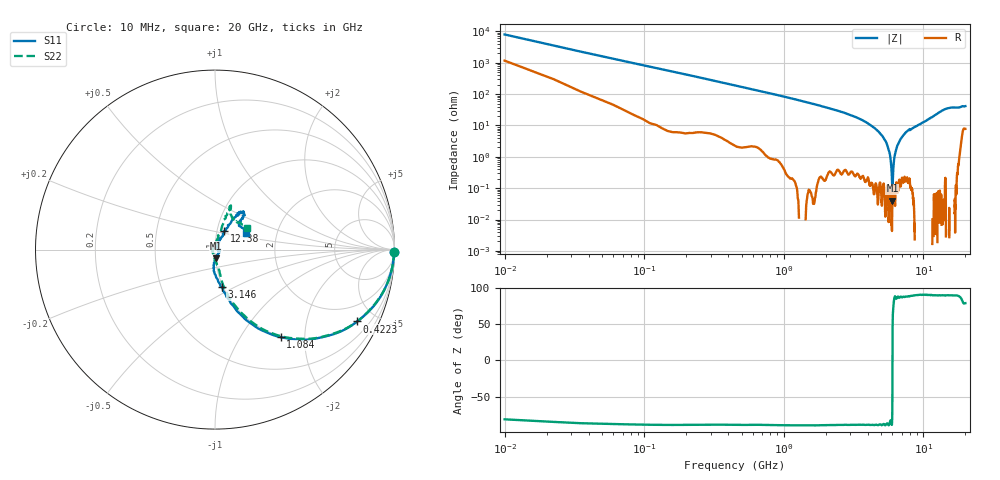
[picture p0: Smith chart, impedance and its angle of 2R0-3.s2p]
!Keysight Technologies,P5008B,MY61100088,A.16.20.02
!Date: Monday, May 27, 2024 14:14:51
!Correction: S11(C  2-Port  )
!S21(C  2-Port  )
!S12(C  2-Port  )
!S22(C  2-Port  )
!S2P File: Measurements: S11, S21, S12, S22:
# Hz S  dB  R 50
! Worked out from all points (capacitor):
!   1601 points, 10 MHz to 20 GHz, reference 50 ohm
!   read as one part in series: C = 1.89 pF near 110 MHz
!   lowest |Z| = 40.3 mohm at 6.007 GHz (marker M1)
!   series resonance near 6.005 GHz, so ESL is about 370 pH
!   S11 on the Smith chart (normalised r, x): 10 MHz: open; 422.3 MHz: 1.04, -3.94; 1.084 GHz: 0.98, -1.52; 3.146 GHz: 0.98, -0.43; 12.38 GHz: 1.08, +0.23; 20 GHz: 1.39, +0.27
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1e7  0.00 -0.7  -38.07 80.9  -38.08 80.9  -0.02 -0.7
1.224438e8  -0.12 -8.4  -16.74 80.7  -16.75 80.7  -0.12 -8.4
1.724188e8  -0.21 -11.8  -14.00 77.6  -14.01 77.6  -0.21 -11.6
4.222938e8  -1.03 -26.8  -7.01 62.6  -7.02 62.6  -1.02 -26.6
1.084462e9  -4.29 -53.1  -2.04 37.1  -2.05 37.1  -4.28 -52.4
1.884062e9  -8.32 -68.8  -0.69 21.6  -0.70 21.6  -8.26 -67.0
3.145931e9  -13.46 -80.2  -0.20 10.1  -0.21 10.2  -13.50 -76.8
3.345831e9  -14.12 -81.8  -0.16 8.9  -0.17 8.9  -14.28 -77.3
6.007e9  -26.16 -86.5  0.01 -2.9  -0.00 -2.8  -26.09 -93.3
6.681662e9  -29.92 -63.2  0.02 -5.0  0.01 -4.9  -30.91 -106.2
7.443781e9  -31.89 -18.5  0.02 -7.1  0.02 -7.1  -37.12 -163.8
7.893556e9  -31.07 -4.8  0.03 -8.3  0.02 -8.3  -36.14 161.3
8.830588e9  -36.44 -7.9  0.04 -10.7  0.03 -10.7  -40.98 151.3
9.530238e9  -38.67 29.4  0.05 -12.5  0.03 -12.4  -39.23 112.7
1.0005e10  -33.74 52.3  0.05 -13.7  0.03 -13.6  -33.97 91.3
1.099201e10  -25.32 64.6  0.04 -16.2  0.03 -16.1  -26.05 78.0
1.237881e10  -18.74 63.6  -0.00 -19.7  -0.01 -19.7  -18.90 72.5
1.334083e10  -14.95 59.6  -0.08 -22.1  -0.09 -22.0  -15.05 72.6
1.499001e10  -11.87 55.4  -0.22 -26.1  -0.23 -26.0  -11.89 70.0
1.667666e10  -12.33 49.8  -0.20 -29.1  -0.21 -29.0  -12.31 69.6
1.832584e10  -14.50 45.1  -0.23 -33.8  -0.24 -33.8  -14.39 55.0
2e10  -14.20 28.2  -0.77 -35.7  -0.78 -35.6  -13.44 34.4
